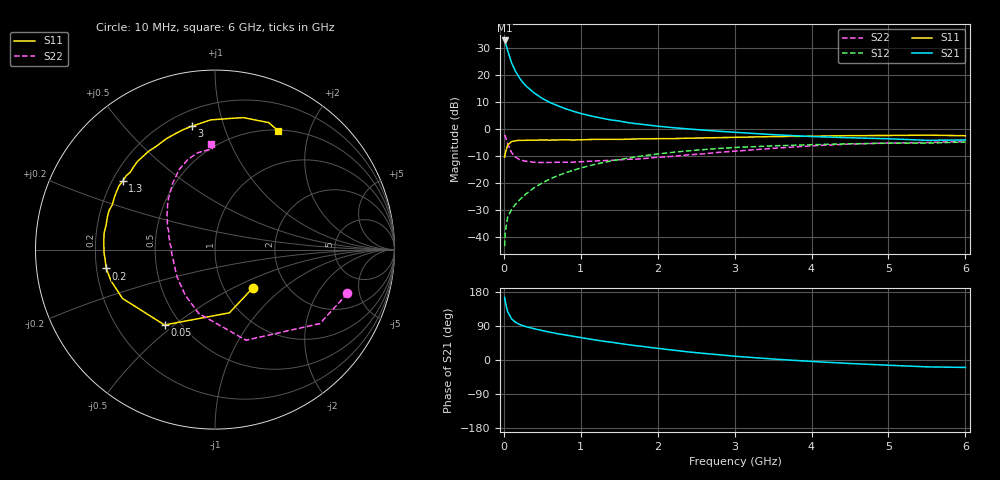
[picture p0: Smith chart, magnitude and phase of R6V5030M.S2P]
! SIEMENS Small Signal Semiconductors
! BFR193
! Si NPN RF Bipolar Junction Transistor in SOT23
! VCE = 0.5 V  IC = 30 mA
! Common Emitter S-Parameters:  May  1996
# GHz  S  MA  R  50
!  f  S11  S21  S12  S22
! GHz  MAG  ANG  MAG  ANG  MAG  ANG  MAG  ANG
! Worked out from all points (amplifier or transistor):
!   36 points, 10 MHz to 6 GHz, reference 50 ohm
!   highest |S21| = 32.7 dB at 10 MHz (marker M1)
!   |S21| within 3 dB of that: start of sweep to 42.67 MHz
!   unconditionally stable (mu >= 1): 276.3 MHz to end of sweep
!   at 250 MHz: K = 0.98, MSG = 21.0 dB, |S12| = -25.0 dB
!   at 1.4 GHz: K = 1.07, MAG = 6.0 dB, |S12| = -11.8 dB
!   at 6 GHz: K = 1.02, MAG = -0.4 dB, |S12| = -4.8 dB
!   S11 on the Smith chart (normalised r, x): 10 MHz: 1.36, -0.64; 50 MHz: 0.41, -0.46; 200 MHz: 0.24, -0.08; 1.3 GHz: 0.24, +0.31; 3 GHz: 0.29, +0.79; 6 GHz: 0.51, +1.54
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0.01  0.3001 -45.3  43.28 165.5  0.0068 75.0  0.7774 -18.3
0.02  0.3613 -77.2  39.84 152.7  0.0128 69.9  0.7151 -35.2
0.05  0.5054 -123.8  28.14 127.5  0.0235 56.3  0.5337 -71.1
0.1  0.5829 -152.2  16.75 108.7  0.0323 53.9  0.3673 -104.3
0.15  0.605 -163.3  11.72 99.8  0.0402 57.4  0.3031 -123.2
0.2  0.6152 -170.2  8.924 94.3  0.0481 60.5  0.2732 -135.0
0.25  0.6149 -175.0  7.146 90.4  0.0565 62.7  0.2598 -144.6
0.3  0.6187 -178.4  6.016 87.3  0.0649 64.4  0.2509 -150.7
0.4  0.6213 175.3  4.578 82.2  0.0827 65.9  0.2417 -159.4
0.5  0.6247 171.5  3.664 77.7  0.1005 66.7  0.2396 -166.4
0.6  0.622 167.0  3.079 73.4  0.1188 66.3  0.2405 -171.3
0.7  0.6263 163.1  2.684 69.4  0.1368 65.3  0.2417 -175.2
0.9  0.6244 156.5  2.126 62.5  0.1719 62.9  0.2432 178.1
1.1  0.6369 149.6  1.782 55.7  0.2067 60.0  0.2523 173.0
1.3  0.6408 143.3  1.553 49.4  0.2404 56.6  0.2596 167.6
1.7  0.6531 131.8  1.26 38.2  0.3012 49.6  0.2765 158.8
2.2  0.6625 119.1  1.056 26.1  0.3704 40.6  0.3115 148.6
3  0.6994 100.7  0.868 10.0  0.4535 26.4  0.3873 131.7
3.5  0.723 91.9  0.785 2.6  0.4869 18.3  0.4385 122.5
4.5  0.7523 77.8  0.687 -9.2  0.5318 4.7  0.5247 106.7
5.5  0.7684 67.1  0.616 -18.1  0.5462 -7.4  0.5617 91.5
6  0.7498 62.1  0.626 -19.6  0.5734 -11.2  0.5862 92.3
